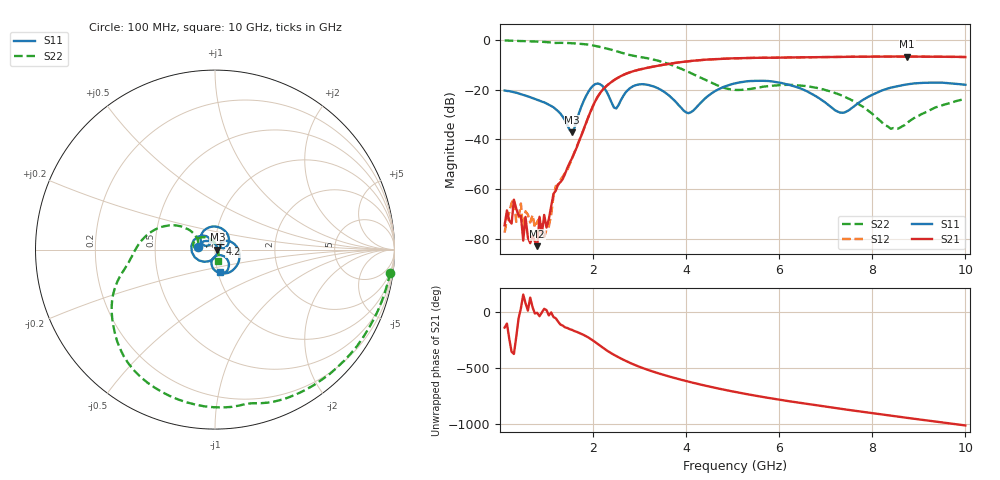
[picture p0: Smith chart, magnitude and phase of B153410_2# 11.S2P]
!  2-Port S-parameters saved by WinCal
! VAR MeasName=S-Parameters (CALIBRATED_DATA) read from VNA (N5245A)
! VAR MeasDate=2016-12-23 9:59:54
! VAR NAME=B153410_2# 11
! VAR FILENAME=B153410_2# 11.S2P
! VAR DATE=2016-12-23 9:59:54
! VAR PHYS_PORTS=1,2
# Hz S DB R 50
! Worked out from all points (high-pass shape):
!   199 points, 100 MHz to 10 GHz, reference 50 ohm
!   highest |S21| = -6.61 dB at 8.75 GHz (marker M1); lowest = -83.1 dB at 800 MHz (marker M2)
!   |S21| within 3 dB of the highest: 3.612 GHz to end of sweep
!   lowest |S11| = -37.1 dB at 1.55 GHz (marker M3), VSWR 1.03, Z = 51.4 + j0.0425 ohm
!   |S11| at or under -10 dB: start of sweep to end of sweep
!   |S22| runs from -35.8 to -0.1 dB; largest |S21 - S12| = 0.0029
!   S11 on the Smith chart (normalised r, x): 100 MHz: 0.83, +0.02; 4.2 GHz: 1.06, +0.06; 10 GHz: 1.03, -0.26
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1e8  -20.32 172.5  -74.65 -137.9  -77.60 106.0  -0.13 -7.5
2.5e8  -20.76 161.3  -73.94 4.5  -65.60 -169.2  -0.25 -17.6
3e8  -21.01 157.5  -64.31 -14.9  -64.04 61.7  -0.28 -21.0
3.5e8  -21.20 154.1  -67.91 138.4  -73.27 18.9  -0.31 -24.3
4.5e8  -21.77 148.1  -70.87 35.0  -65.86 -75.2  -0.37 -30.9
5e8  -22.07 145.1  -80.83 159.0  -77.42 94.0  -0.38 -34.2
5.5e8  -22.37 142.3  -71.27 80.3  -69.03 17.6  -0.42 -37.6
8e8  -24.06 130.0  -83.06 -5.1  -73.17 -176.5  -0.59 -53.9
9.5e8  -25.09 121.9  -70.46 31.1  -79.39 -9.9  -0.73 -63.7
1e9  -25.53 119.0  -75.55 19.7  -76.40 -25.2  -0.79 -67.1
1.2e9  -27.85 103.0  -60.66 -54.5  -58.84 -53.2  -1.15 -78.5
1.55e9  -37.12 1.7  -47.53 -159.0  -47.78 -160.3  -1.25 -100.4
1.75e9  -26.72 -94.3  -38.41 165.6  -38.43 164.9  -1.52 -113.5
2.3e9  -21.07 122.2  -18.30 15.2  -18.29 15.4  -3.42 -148.5
3.4e9  -19.46 46.3  -10.31 171.8  -10.30 172.0  -8.31 167.2
4.2e9  -27.53 44.9  -8.23 81.1  -8.22 81.1  -14.12 143.3
5.05e9  -17.43 -5.3  -7.32 4.2  -7.33 4.4  -20.06 161.9
6.7e9  -21.66 -103.7  -6.88 -110.2  -6.88 -110.2  -18.88 146.5
7.35e9  -29.29 -71.1  -6.76 -149.2  -6.75 -149.2  -22.35 121.0
8.35e9  -19.41 -44.0  -6.64 153.4  -6.62 153.6  -35.03 38.1
8.75e9  -17.83 -54.6  -6.61 131.1  -6.62 131.2  -33.35 -32.2
1e10  -18.00 -77.2  -6.82 62.8  -6.82 63.1  -23.67 -75.5
